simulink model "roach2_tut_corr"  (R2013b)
settings: Solver=VariableStepDiscrete  SolverMode=SingleTasking  StartTime=0.0  StopTime=100  RelTol=1e-3
undefined symbols (not defined in the file): add_latency, addr_width, Bit, bitfield, BitWidth, bram_latency, burst_size, casper_library_scopes, conv_latency, data_width, DelayLen, fan_latency, FFTSize, FFTStage, getfield, increment, led, Location, Lower, mult_latency, mux_latency, n_bits, n_bits_data, n_inputs, n_streams, n_taps, neg_latency, negate_latency, nsamples, pfb_size, pulse_len, reset_period, ROACH, ROACH2, snapshot, sx475t, sync_period, sync_period_bits, Upper, UseCounter, Width
libraries: xbsIndex_r4 x24444, casper_library_misc x73, xbsReplacements_r4 x34, casper_library_delays x14, xps_library x7
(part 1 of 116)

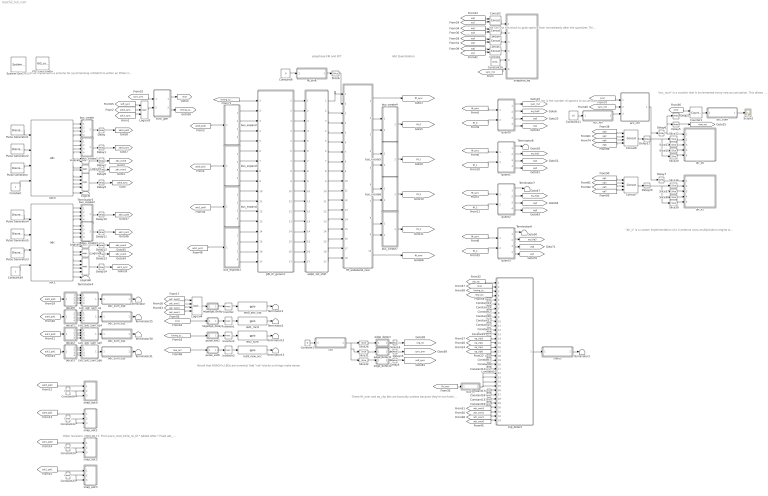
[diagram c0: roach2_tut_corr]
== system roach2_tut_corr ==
  note: This circuit implements a scheme for synchronizing a ROACH to within an FPGA clock of a second boundary using an external 1 pulse-per-second device. * A sync_arm command will cause the sync_gen to stop issuing sync pulses. * It will then ignore the next input trigger (1PPS), while sync is flushed through the DSP pipeline. * It will then lock onto the next trigger (1PPS) and issue syncs thereafter every sync_period clocks. * Need a multiple of (pfb_fir taps*LCM(FFT reorder orders) *fft bins/parallel inputs =) (4 * LCM(2,2,2,9) * 1024 / 4) = 18432) for sync_period for simulation * Trigger off either ADC's 1PPS inputs
  note: polyphase FIR and FFT
  note: "dir_x" is a custom implementation of a 4 antenna cross-multiplication engine which uses a multiplication core for each auto- and cross-correlation. Some BRAM space is wasted in this 1024 channel compile because the minimum shared BRAM size is 2048.
  note: "acc_num" is a counter that is incremented every new accumulation. This allows a computer to know when a new accumulation is available.
  note: acc_len is the number of spectra to accumulate.
  note: 4bit Quantisation
  note: Recall that ROACH's LEDs are inverted. Add "not" blocks so things make sense.
  note: Older revisions: 2009-08-17: From poco_mod_1024_no_fd * Added LEDs * Fixed adc_levels 2009-08-18: r310 * Changed dir_x numbering scheme * mods to adc_levels * added status register * EQ now per channel 2010-08-14: r313 * adc_sum_sq copied from kat-7 feng 2010-08-16: r314: * tidyup for workshop 2012-05-09: r315: * replaced FFT and PFB_FIR with new library ones * software register replacement 2013-08-16: r316: Updated for workshop. Ran DM's update_casper_blocks script Replaced all cross-multiplication modules with dsp48_cmults Replaced deprecated snap blocks Replaced FFT and FIR blocks for combined multi-input blocks.
  note: These fft_over and eq_clip bits are basically useless because they're non-latching. The chances of catching an actual overrange event from software is pretty small, unless they're continuously overranging.
  note: We can use this block to grab spectra from immediately after the quantizer. This will help determine what the correct quantizer EQ coefficients are
  " System Generator" : xbsIndex_r4/ System Generator  Tag=genX  xilinxfamily=virtex6  part=xc6vsx475t  speed=-1  package=ff1759  synthesis_tool=XST  clock_wrapper=Clock Enables  directory=./roach2_tut_corr/sysgen  proj_type=Project Navigator  Synth_file=XST Defaults  Impl_file=ISE Defaults  testbench=off  simulink_period=1  sysclk_period=5  dcm_input_clock_period=100  incr_netlist=off  trim_vbits=Everywhere in SubSystem  dbl_ovrd=According to Block Masks  core_generation=According to Block Masks  run_coregen=off  deprecated_control=off  eval_field=0  block_type=sysgen
  Concat{1..4} (4 alike) : xbsIndex_r4/Concat  num_inputs=2  dbl_ovrd=off  block_type=concat
  Concat6 : xbsIndex_r4/Concat  num_inputs=4  dbl_ovrd=off  block_type=concat
  Concat7 : xbsIndex_r4/Concat  num_inputs=4  dbl_ovrd=off  block_type=concat
  Constant : Constant  SampleTime=1/4
  Constant1 : Constant  Value=0
  Constant{2..5,7..8,10,12..21} (17 alike) : xbsIndex_r4/Constant  const=0  gui_display_data_type=Fixed-point  arith_type=Boolean  n_bits=1  bin_pt=0  preci_type=Single  exp_width=8  frac_width=24  explicit_period=on  period=1  equ=P=C  opselect=C  inp2=PCIN>>17  opr=+  inp1=P  carry=CIN  dbl_ovrd=off  block_type=constant
  Constant11 : Constant  Value=10
  Constant{6,22..24} (4 alike) : xbsIndex_r4/Constant  const=1  gui_display_data_type=Boolean  arith_type=Boolean  n_bits=16  bin_pt=14  preci_type=Single  exp_width=8  frac_width=24  explicit_period=on  period=1  equ=P=C  opselect=C  inp2=PCIN>>17  opr=+  inp1=P  carry=CIN  dbl_ovrd=off  block_type=constant
  Constant26 : xbsIndex_r4/Constant  const=0  gui_display_data_type=Boolean  arith_type=Boolean  n_bits=32  bin_pt=0  preci_type=Single  exp_width=8  frac_width=24  explicit_period=on  period=1  equ=P=C  opselect=C  inp2=PCIN>>17  opr=+  inp1=P  carry=CIN  dbl_ovrd=off  block_type=constant
  Constant39 : Constant  SampleTime=1/4
  Constant9 : Constant  Value=0
  Counter1 : xbsIndex_r4/Counter  cnt_type=Free Running  cnt_to=Inf  operation=Up  start_count=0  cnt_by_val=1  arith_type=Unsigned  n_bits=32  bin_pt=0  load_pin=off  rst=on  en=on  explicit_period=off  period=1  dbl_ovrd=off  use_behavioral_HDL=off  implementation=Fabric  use_rpm=on  block_type=counter
  Delay{,1..2,4..16} (16 alike) : xbsIndex_r4/Delay  rst=off  infoeditControl=Selection of Reset will increase slice count due to use of real FFs and instead of SRLs  en=off  latency=1  dbl_ovrd=off  reg_retiming=on  block_type=delay
  Delay20 : xbsIndex_r4/Delay  rst=off  infoeditControl=Selection of Reset will increase slice count due to use of real FFs and instead of SRLs  en=off  latency=2  dbl_ovrd=off  reg_retiming=on  block_type=delay
  Delay21 : xbsIndex_r4/Delay  rst=off  infoeditControl=Selection of Reset will increase slice count due to use of real FFs and instead of SRLs  en=off  latency=2  dbl_ovrd=off  reg_retiming=on  block_type=delay
  Delay3 : xbsIndex_r4/Delay  rst=off  infoeditControl=Selection of Reset will increase slice count due to use of real FFs and instead of SRLs  en=off  latency=2  dbl_ovrd=off  reg_retiming=on  block_type=delay
  Inverter{,1..3} (4 alike) : xbsIndex_r4/Inverter  en=off  latency=1  dbl_ovrd=off  block_type=inv
  Logical : xbsIndex_r4/Logical  logical_function=OR  inputs=4  en=off  latency=0  precision=Full  arith_type=Unsigned  n_bits=16  bin_pt=0  align_bp=on  dbl_ovrd=off  block_type=logical
  Logical{1..2,8..9} (4 alike) : xbsIndex_r4/Logical  logical_function=OR  inputs=2  en=off  latency=0  precision=Full  arith_type=Unsigned  n_bits=16  bin_pt=0  align_bp=on  dbl_ovrd=off  block_type=logical
  Logical3 : xbsIndex_r4/Logical  logical_function=OR  inputs=3  en=off  latency=0  precision=Full  arith_type=Unsigned  n_bits=16  bin_pt=0  align_bp=on  dbl_ovrd=off  block_type=logical
  Logical4 : xbsIndex_r4/Logical  logical_function=OR  inputs=4  en=off  latency=0  precision=Full  arith_type=Unsigned  n_bits=8  bin_pt=2  align_bp=on  dbl_ovrd=off  block_type=logical
  Logical6 : xbsIndex_r4/Logical  logical_function=OR  inputs=4  en=off  latency=0  precision=Full  arith_type=Unsigned  n_bits=16  bin_pt=0  align_bp=on  dbl_ovrd=off  block_type=logical
  Pulse Generator : DiscretePulseGenerator  Period=2^8  PhaseDelay=11  SampleTime=1/4
  Pulse Generator1 : DiscretePulseGenerator  Amplitude=0.75  Period=2^10  PhaseDelay=9+13+2^8  SampleTime=1/4
  Pulse Generator2 : DiscretePulseGenerator  Amplitude=0.5  Period=2^10  PhaseDelay=9+14+2^8  SampleTime=1/4
  Pulse Generator3 : DiscretePulseGenerator  Period=2^8  PhaseDelay=11  SampleTime=1/4
  Pulse Generator4 : DiscretePulseGenerator  Amplitude=0.75  Period=2^14  PhaseDelay=23+2^8  SampleTime=1/4
  Pulse Generator5 : DiscretePulseGenerator  Amplitude=0.5  Period=2^14  PhaseDelay=22+2^8  SampleTime=1/4
  Scope2 : Scope
  Slice12 : xbsIndex_r4/Slice  nbits=8  boolean_output=off  mode=Lower Bit Location + Width  bit1=0  base1=MSB of Input  bit0=24  base0=LSB of Input  dbl_ovrd=off  block_type=slice
  Slice13 : xbsIndex_r4/Slice  nbits=8  boolean_output=off  mode=Lower Bit Location + Width  bit1=0  base1=MSB of Input  bit0=16  base0=LSB of Input  dbl_ovrd=off  block_type=slice
  Slice15 : xbsIndex_r4/Slice  nbits=8  boolean_output=off  mode=Lower Bit Location + Width  bit1=0  base1=MSB of Input  bit0=8  base0=LSB of Input  dbl_ovrd=off  block_type=slice
  Slice20 : xbsIndex_r4/Slice  nbits=8  boolean_output=off  mode=Lower Bit Location + Width  bit1=0  base1=MSB of Input  bit0=0  base0=LSB of Input  dbl_ovrd=off  block_type=slice
  Slice26 : xbsIndex_r4/Slice  nbits=1  boolean_output=on  mode=Lower Bit Location + Width  bit1=0  base1=MSB of Input  bit0=16  base0=LSB of Input  dbl_ovrd=off  block_type=slice
  Slice31 : xbsIndex_r4/Slice  nbits=1  boolean_output=on  mode=Lower Bit Location + Width  bit1=0  base1=MSB of Input  bit0=17  base0=LSB of Input  dbl_ovrd=off  block_type=slice
  Slice32 : xbsIndex_r4/Slice  nbits=1  boolean_output=on  mode=Lower Bit Location + Width  bit1=0  base1=MSB of Input  bit0=18  base0=LSB of Input  dbl_ovrd=off  block_type=slice
  Slice36 : xbsIndex_r4/Slice  nbits=8  boolean_output=off  mode=Lower Bit Location + Width  bit1=0  base1=MSB of Input  bit0=24  base0=LSB of Input  dbl_ovrd=off  block_type=slice
  Slice37 : xbsIndex_r4/Slice  nbits=8  boolean_output=off  mode=Lower Bit Location + Width  bit1=0  base1=MSB of Input  bit0=16  base0=LSB of Input  dbl_ovrd=off  block_type=slice
  Slice38 : xbsIndex_r4/Slice  nbits=8  boolean_output=off  mode=Lower Bit Location + Width  bit1=0  base1=MSB of Input  bit0=8  base0=LSB of Input  dbl_ovrd=off  block_type=slice
  Slice39 : xbsIndex_r4/Slice  nbits=8  boolean_output=off  mode=Lower Bit Location + Width  bit1=0  base1=MSB of Input  bit0=0  base0=LSB of Input  dbl_ovrd=off  block_type=slice
  Slice6 : xbsIndex_r4/Slice  nbits=11  boolean_output=off  mode=Lower Bit Location + Width  bit1=0  base1=MSB of Input  bit0=0  base0=LSB of Input  dbl_ovrd=off  block_type=slice
  Terminator{,1..8,12..13,25,30..31} (14 alike) : Terminator
  XSG core config : xps_library/XSG_core_config  Tag=xps:xsg  hw_sys=ROACH2:sx475t  clk_src=adc0_clk  ROACH_clk_src=adc0_clk  ROACH2_clk_src=adc0_clk  MKDIG_clk_src=sys_clk  clk_rate=200  sample_period=1  synthesis_tool=XST
  a0p0_1st_shift : Subsystem
  acc_ctrl : Subsystem
  acc_len : Subsystem  Tag=xps:sw_reg  AncestorBlock=xps_library/software_register
  acc_num : Subsystem  Tag=xps:sw_reg  AncestorBlock=xps_library/software_register
  adc0 : xps_library/ADCs/adc  Tag=xps:adc  adc_brd=adc0  adc_clk_rate=800  adc_interleave=off  sample_period=1
  adc1 : xps_library/ADCs/adc  Tag=xps:adc  adc_brd=adc1  adc_clk_rate=800  adc_interleave=off  sample_period=1
  adc_sum_sq0 : Subsystem  Tag=xps:sw_reg  AncestorBlock=xps_library/software_register
  adc_sum_sq1 : Subsystem  Tag=xps:sw_reg  AncestorBlock=xps_library/software_register
  adc_sum_sq2 : Subsystem  Tag=xps:sw_reg  AncestorBlock=xps_library/software_register
  adc_sum_sq3 : Subsystem  Tag=xps:sw_reg  AncestorBlock=xps_library/software_register
  bus_create : Subsystem  AncestorBlock=casper_library_flow_control/bus_create
  bus_create1 : Subsystem  AncestorBlock=casper_library_flow_control/bus_create
  bus_create2 : Subsystem  AncestorBlock=casper_library_flow_control/bus_create
  bus_create3 : Subsystem  AncestorBlock=casper_library_flow_control/bus_create
  bus_create4 : Subsystem  AncestorBlock=casper_library_flow_control/bus_create
  bus_create5 : Subsystem  AncestorBlock=casper_library_flow_control/bus_create
  bus_create6 : Subsystem  AncestorBlock=casper_library_flow_control/bus_create
  bus_create7 : Subsystem  AncestorBlock=casper_library_flow_control/bus_create
  bus_expand : Subsystem  AncestorBlock=casper_library_flow_control/bus_expand
  bus_expand1 : Subsystem  AncestorBlock=casper_library_flow_control/bus_expand
  bus_expand2 : Subsystem  AncestorBlock=casper_library_flow_control/bus_expand
  bus_expand3 : Subsystem  AncestorBlock=casper_library_flow_control/bus_expand
  bus_or : Subsystem
  calc_adc_sum_sq : Subsystem
  calc_adc_sum_sq4 : Subsystem
  calc_adc_sum_sq5 : Subsystem
  calc_adc_sum_sq6 : Subsystem
  clip_detect : Subsystem
  ctrl : Subsystem  Tag=xps:sw_reg  AncestorBlock=xps_library/software_register
  decat0 : Subsystem
  decat1 : Subsystem
  decat2 : Subsystem
  decat3 : Subsystem
  dir_x0 : Subsystem
  dir_x1 : Subsystem
  edge_detect : Subsystem  AncestorBlock=casper_library_misc/edge_detect
  edge_detect1 : Subsystem  AncestorBlock=casper_library_misc/edge_detect
  edge_detect2 : Subsystem  AncestorBlock=casper_library_misc/edge_detect
  fft_shift : Subsystem  Tag=xps:sw_reg  AncestorBlock=xps_library/software_register
  fft_wideband_real : Subsystem  Tag=casper:fft_wideband_real  AncestorBlock=casper_library_ffts/fft_wideband_real
  led0_adc_clip : xps_library/gpio  Tag=xps:gpio  io_group=ROACH:led  io_dir=out  arith_type=Boolean  bitwidth=1  bin_pt=0  bit_index=0  sample_period=1  use_single_ended=off  use_ddr=off  reg_iob=on  reg_clk_phase=0  termination=None
  led1_mrst : xps_library/gpio  Tag=xps:gpio  io_group=ROACH:led  io_dir=out  arith_type=Boolean  bitwidth=1  bin_pt=0  bit_index=1  sample_period=1  use_single_ended=off  use_ddr=off  reg_iob=on  reg_clk_phase=0  termination=None
  led2_sync : xps_library/gpio  Tag=xps:gpio  io_group=ROACH:led  io_dir=out  arith_type=Boolean  bitwidth=1  bin_pt=0  bit_index=2  sample_period=1  use_single_ended=off  use_ddr=off  reg_iob=on  reg_clk_phase=0  termination=None
  led3_new_acc : xps_library/gpio  Tag=xps:gpio  io_group=ROACH:led  io_dir=out  arith_type=Unsigned  bitwidth=1  bin_pt=0  bit_index=3  sample_period=1  use_single_ended=off  use_ddr=off  reg_iob=on  reg_clk_phase=0  termination=None
  negedge_delay : Subsystem  AncestorBlock=casper_library_misc/negedge_delay
  negedge_delay1 : Subsystem  AncestorBlock=casper_library_misc/negedge_delay
  pfb_fir_generic : Subsystem  Tag=casper:pfb_fir_generic  AncestorBlock=casper_library_pfbs/pfb_fir_generic
  pulse_ext2 : Subsystem
  pulse_ext6 : Subsystem
  quant0 : Subsystem
  quant1 : Subsystem
  quant2 : Subsystem
  quant3 : Subsystem
  snap_adc0 : Subsystem  Tag=casper:snapshot  AncestorBlock=casper_library_scopes/snapshot
  snap_adc1 : Subsystem  Tag=casper:snapshot  AncestorBlock=casper_library_scopes/snapshot
  snap_adc2 : Subsystem  Tag=casper:snapshot  AncestorBlock=casper_library_scopes/snapshot
  snap_adc3 : Subsystem  Tag=casper:snapshot  AncestorBlock=casper_library_scopes/snapshot
  snapshot_eq : Subsystem  Tag=casper:bitsnap  AncestorBlock=casper_library_scopes/bitfield snapshot
  status : Subsystem  Tag=xps:sw_reg  AncestorBlock=xps_library/software_register
  sync_gen : Subsystem
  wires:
  adc0/16 -> Logical/4
  adc0/15 -> Logical/3
  adc0/14 -> Logical/2
  adc0/13 -> Logical/1
  Logical/1 -> Delay9/1
  adc0/9 -> Logical2/1
  adc0/10 -> Logical2/2
  adc0/11 -> Logical1/1
  adc0/12 -> Logical1/2
  Logical2/1 -> Delay2/1
  adc0/5 -> bus_create1/1(in1)
  adc0/6 -> bus_create1/2(in2)
  adc0/7 -> bus_create1/3(in3)
  adc0/8 -> bus_create1/4(in4)
  bus_create1/1(bus_out) -> Delay1/1
  adc0/1 -> bus_create/1(in1)
  adc0/2 -> bus_create/2(in2)
  adc0/3 -> bus_create/3(in3)
  adc0/4 -> bus_create/4(in4)
  bus_create/1(bus_out) -> Delay/1
  Pulse Generator/1 -> adc0/3
  Pulse Generator1/1 -> adc0/1
  Pulse Generator2/1 -> adc0/2
  Constant/1 -> adc0/4
  [adc0_sync] -> Logical3/2
  sync_gen/1(mrst) -> [mrst]
  sync_gen/2(sync) -> [timing_sync]
  Logical3/1 -> sync_gen/2(pps)
  [soft_sync] -> Logical3/1
  Constant9/1 -> fft_shift/1(sim_1)
  fft_shift/1(in_reg) -> Slice6/1
  [adc0_pol0] -> bus_expand/1(bus_in)
  adc1/16 -> Logical6/4
  adc1/15 -> Logical6/3
  adc1/14 -> Logical6/2
  adc1/13 -> Logical6/1
  Logical6/1 -> Delay14/1
  Pulse Generator3/1 -> adc1/3
  Pulse Generator4/1 -> adc1/1
  Pulse Generator5/1 -> adc1/2
  Constant39/1 -> adc1/4
  Logical1/1 -> Delay8/1
  quant0/1(sync_out) -> [sync_rnd]
  quant0/3(dout0) -> [eq0]
  quant0/4(dout1) -> [eq1]
  Constant11/1 -> acc_len/1(sim_1)
  acc_len/1(in_reg) -> acc_ctrl/3(acc_len)
  Concat6/1 -> Delay21/1
  Slice12/1 -> dir_x0/2(a)
  Slice13/1 -> dir_x0/3(b)
  Slice15/1 -> dir_x0/4(c)
  Slice20/1 -> dir_x0/5(d)
  Counter1/1 -> acc_num/1(out_reg)
  acc_ctrl/1(new_acc) -> Delay6/1, Delay7/1
  [mrst] -> acc_ctrl/1(mrst)
  Delay5/1 -> [new_acc]
  [sync_rnd] -> acc_ctrl/2(sync)
  acc_num/1(sim_out) -> Scope2/1
  Delay3/1 -> Counter1/2
  [mrst] -> Counter1/1
  Delay6/1 -> dir_x0/1(new_acc), Delay3/1, Delay5/1
  [eq0] -> Concat6/1
  [eq2] -> Concat6/2
  [eq4] -> Concat6/3
  [eq6] -> Concat6/4
  [eq1] -> Concat7/1
  [eq3] -> Concat7/2
  [eq5] -> Concat7/3
  [eq7] -> Concat7/4
  Delay20/1 -> Slice37/1, Slice38/1, Slice39/1, Slice36/1
  Slice36/1 -> dir_x1/2(a)
  Slice37/1 -> dir_x1/3(b)
  Slice38/1 -> dir_x1/4(c)
  Slice39/1 -> dir_x1/5(d)
  Concat7/1 -> Delay20/1
  Delay7/1 -> dir_x1/1(new_acc)
  [adc1_sync] -> Logical3/3
  Constant1/1 -> ctrl/1(sim_1)
  ctrl/1(in_reg) -> Slice26/1, Slice31/1, Slice32/1
  adc0/17 -> Terminator5/1
  adc1/17 -> Terminator4/1
  [clip_rst] -> clip_detect/1(rst)
  [adc_over3] -> clip_detect/30(In_03)
  [adc_over2] -> clip_detect/31(In_02)
  [adc_over1] -> clip_detect/32(In_01)
  [adc_over0] -> clip_detect/33(in_lsb)
  Constant16/1 -> clip_detect/29(In_04)
  Constant17/1 -> clip_detect/26(In_07)
  Constant18/1 -> clip_detect/27(In_06)
  Constant13/1 -> clip_detect/28(In_05)
  [mrst] -> clip_detect/2(in_msb_nr)
  [timing_sync] -> clip_detect/3(In_30_nr)
  [new_acc] -> clip_detect/4(In_29_nr)
  Constant14/1 -> clip_detect/5(In_28_nr)
  Constant19/1 -> clip_detect/6(In_27_nr)
  Constant2/1 -> clip_detect/7(In_26_nr)
  Constant20/1 -> clip_detect/8(In_25_nr)
  Constant21/1 -> clip_detect/9(In_24_nr)
  [eq_clip3] -> clip_detect/14(In_19)
  [eq_clip2] -> clip_detect/15(In_18)
  [eq_clip1] -> clip_detect/16(In_17)
  [eq_clip0] -> clip_detect/17(In_16)
  Constant7/1 -> clip_detect/18(In_15)
  Constant8/1 -> clip_detect/19(In_14)
  Constant10/1 -> clip_detect/20(In_13)
  Constant12/1 -> clip_detect/21(In_12)
  clip_detect/1(registered_out) -> status/1(out_reg)
  Slice26/1 -> edge_detect/1(in)
  [adc0_pol0] -> decat0/1(In1)
  Slice31/1 -> edge_detect1/1(in)
  Slice32/1 -> edge_detect2/1(in)
  edge_detect1/1(out) -> Delay15/1
  edge_detect/1(out) -> Delay16/1
  edge_detect2/1(out) -> Delay4/1
  [sync_arm] -> sync_gen/1(arm)
  Delay/1 -> [adc0_pol0]
  Delay1/1 -> [adc0_pol1]
  Delay2/1 -> [adc_over0]
  Delay8/1 -> [adc_over1]
  Delay9/1 -> [adc0_sync]
  Delay10/1 -> [adc1_pol0]
  Delay11/1 -> [adc1_pol1]
  Delay12/1 -> [adc_over2]
  Delay13/1 -> [adc_over3]
  Delay14/1 -> [adc1_sync]
  Delay21/1 -> Slice12/1, Slice13/1, Slice15/1, Slice20/1
  pulse_ext2/1(out) -> Inverter2/1
  [timing_sync] -> pulse_ext2/1(in)
  [mrst] -> negedge_delay1/1(in)
  pulse_ext6/1(out) -> Inverter3/1
  [new_acc] -> pulse_ext6/1(in)
  led0_adc_clip/1 -> Terminator1/1
  led1_mrst/1 -> Terminator2/1
  led2_sync/1 -> Terminator12/1
  led3_new_acc/1 -> Terminator13/1
  Logical4/1 -> negedge_delay/1(in)
  negedge_delay/1(out) -> Inverter/1
  [adc_over0] -> Logical4/1
  [adc_over1] -> Logical4/2
  [adc_over2] -> Logical4/3
  [adc_over3] -> Logical4/4
  negedge_delay1/1(out) -> Inverter1/1
  status/1(sim_out) -> Terminator3/1
  Constant15/1 -> clip_detect/10(In_23)
  Constant3/1 -> clip_detect/11(In_22)
  Constant4/1 -> clip_detect/12(In_21)
  Constant5/1 -> clip_detect/13(In_20)
  quant0/2(clip_out) -> [eq_clip0]
  quant1/1(sync_out) -> Terminator8/1
  quant1/3(dout0) -> [eq2]
  quant1/4(dout1) -> [eq3]
  quant1/2(clip_out) -> [eq_clip1]
  quant2/1(sync_out) -> Terminator7/1
  quant2/3(dout0) -> [eq4]
  quant2/2(clip_out) -> [eq_clip2]
  quant3/1(sync_out) -> Terminator6/1
  quant3/3(dout0) -> [eq6]
  quant3/4(dout1) -> [eq7]
  quant3/2(clip_out) -> [eq_clip3]
  Delay4/1 -> [soft_sync]
  Delay15/1 -> [sync_arm]
  Delay16/1 -> [clip_rst]
  Inverter/1 -> led0_adc_clip/1
  Inverter1/1 -> led1_mrst/1
  Inverter2/1 -> led2_sync/1
  Inverter3/1 -> led3_new_acc/1
  adc1/9 -> Logical9/1
  adc1/10 -> Logical9/2
  adc1/11 -> Logical8/1
  adc1/12 -> Logical8/2
  Logical9/1 -> Delay12/1
  Logical8/1 -> Delay13/1
  adc1/5 -> bus_create3/1(in1)
  adc1/6 -> bus_create3/2(in2)
  adc1/7 -> bus_create3/3(in3)
  adc1/8 -> bus_create3/4(in4)
  bus_create3/1(bus_out) -> Delay11/1
  adc1/1 -> bus_create2/1(in1)
  adc1/2 -> bus_create2/2(in2)
  adc1/3 -> bus_create2/3(in3)
  adc1/4 -> bus_create2/4(in4)
  bus_create2/1(bus_out) -> Delay10/1
  calc_adc_sum_sq/1(sum_sq) -> adc_sum_sq0/1(out_reg)
  decat0/1(Out1) -> calc_adc_sum_sq/1(In1)
  decat0/2(Out2) -> calc_adc_sum_sq/2(In2)
  decat0/3(Out3) -> calc_adc_sum_sq/3(In3)
  decat0/4(Out4) -> calc_adc_sum_sq/4(In4)
  adc_sum_sq0/1(sim_out) -> Terminator/1
  calc_adc_sum_sq4/1(sum_sq) -> adc_sum_sq1/1(out_reg)
  decat1/1(Out1) -> calc_adc_sum_sq4/1(In1)
  decat1/2(Out2) -> calc_adc_sum_sq4/2(In2)
  decat1/3(Out3) -> calc_adc_sum_sq4/3(In3)
  decat1/4(Out4) -> calc_adc_sum_sq4/4(In4)
  adc_sum_sq1/1(sim_out) -> Terminator25/1
  calc_adc_sum_sq5/1(sum_sq) -> adc_sum_sq2/1(out_reg)
  decat2/1(Out1) -> calc_adc_sum_sq5/1(In1)
  decat2/2(Out2) -> calc_adc_sum_sq5/2(In2)
  decat2/3(Out3) -> calc_adc_sum_sq5/3(In3)
  decat2/4(Out4) -> calc_adc_sum_sq5/4(In4)
  adc_sum_sq2/1(sim_out) -> Terminator30/1
  calc_adc_sum_sq6/1(sum_sq) -> adc_sum_sq3/1(out_reg)
  decat3/1(Out1) -> calc_adc_sum_sq6/1(In1)
  decat3/2(Out2) -> calc_adc_sum_sq6/2(In2)
  decat3/3(Out3) -> calc_adc_sum_sq6/3(In3)
  decat3/4(Out4) -> calc_adc_sum_sq6/4(In4)
  adc_sum_sq3/1(sim_out) -> Terminator31/1
  [adc0_pol1] -> decat1/1(In1)
  [adc1_pol0] -> decat2/1(In1)
  [adc1_pol1] -> decat3/1(In1)
  quant2/4(dout1) -> [eq5]
  [fft_over] -> bus_or/1(In1)
  Slice6/1 -> fft_wideband_real/2(shift)
  fft_wideband_real/10(of) -> [fft_over]
  a0p0_1st_shift/1(sync_out) -> fft_wideband_real/1(sync)
  a0p0_1st_shift/14(dout13) -> fft_wideband_real/15(in30)
  a0p0_1st_shift/10(dout9) -> fft_wideband_real/11(in20)
  a0p0_1st_shift/11(dout10) -> fft_wideband_real/12(in21)
  a0p0_1st_shift/12(dout11) -> fft_wideband_real/13(in22)
  a0p0_1st_shift/13(dout12) -> fft_wideband_real/14(in23)
  a0p0_1st_shift/15(dout14) -> fft_wideband_real/16(in31)
  a0p0_1st_shift/16(dout15) -> fft_wideband_real/17(in32)
  a0p0_1st_shift/17(dout16) -> fft_wideband_real/18(in33)
  a0p0_1st_shift/6(dout5) -> fft_wideband_real/7(in10)
  a0p0_1st_shift/7(dout6) -> fft_wideband_real/8(in11)
  a0p0_1st_shift/8(dout7) -> fft_wideband_real/9(in12)
  a0p0_1st_shift/9(dout8) -> fft_wideband_real/10(in13)
  a0p0_1st_shift/2(dout1) -> fft_wideband_real/3(in00)
  a0p0_1st_shift/3(dout2) -> fft_wideband_real/4(in01)
  a0p0_1st_shift/5(dout4) -> fft_wideband_real/6(in03)
  a0p0_1st_shift/4(dout3) -> fft_wideband_real/5(in02)
  [adc0_pol1] -> bus_expand1/1(bus_in)
  [adc1_pol0] -> bus_expand2/1(bus_in)
  [adc1_pol1] -> bus_expand3/1(bus_in)
  pfb_fir_generic/1(sync_out) -> a0p0_1st_shift/1(sync_in)
  pfb_fir_generic/2(pol0_out0) -> a0p0_1st_shift/2(din1)
  pfb_fir_generic/6(pol1_out0) -> a0p0_1st_shift/6(din5)
  pfb_fir_generic/7(pol1_out1) -> a0p0_1st_shift/7(din6)
  pfb_fir_generic/8(pol1_out2) -> a0p0_1st_shift/8(din7)
  pfb_fir_generic/14(pol3_out0) -> a0p0_1st_shift/14(din13)
  pfb_fir_generic/3(pol0_out1) -> a0p0_1st_shift/3(din2)
  pfb_fir_generic/5(pol0_out3) -> a0p0_1st_shift/5(din4)
  pfb_fir_generic/10(pol2_out0) -> a0p0_1st_shift/10(din9)
  pfb_fir_generic/13(pol2_out3) -> a0p0_1st_shift/13(din12)
  pfb_fir_generic/15(pol3_out1) -> a0p0_1st_shift/15(din14)
  pfb_fir_generic/12(pol2_out2) -> a0p0_1st_shift/12(din11)
  pfb_fir_generic/4(pol0_out2) -> a0p0_1st_shift/4(din3)
  pfb_fir_generic/11(pol2_out1) -> a0p0_1st_shift/11(din10)
  pfb_fir_generic/16(pol3_out2) -> a0p0_1st_shift/16(din15)
  pfb_fir_generic/17(pol3_out3) -> a0p0_1st_shift/17(din16)
  pfb_fir_generic/9(pol1_out3) -> a0p0_1st_shift/9(din8)
  [timing_sync] -> pfb_fir_generic/1(sync)
  bus_expand/2(out3) -> pfb_fir_generic/3(pol0_in1)
  bus_expand/3(out2) -> pfb_fir_generic/4(pol0_in2)
  bus_expand/4(lsb_out1) -> pfb_fir_generic/5(pol0_in3)
  bus_expand/1(msb_out4) -> pfb_fir_generic/2(pol0_in0)
  bus_expand1/1(msb_out4) -> pfb_fir_generic/6(pol1_in0)
  bus_expand1/2(out3) -> pfb_fir_generic/7(pol1_in1)
  bus_expand1/3(out2) -> pfb_fir_generic/8(pol1_in2)
  bus_expand1/4(lsb_out1) -> pfb_fir_generic/9(pol1_in3)
  bus_expand2/2(out3) -> pfb_fir_generic/11(pol2_in1)
  bus_expand2/3(out2) -> pfb_fir_generic/12(pol2_in2)
  bus_expand2/4(lsb_out1) -> pfb_fir_generic/13(pol2_in3)
  bus_expand2/1(msb_out4) -> pfb_fir_generic/10(pol2_in0)
  bus_expand3/2(out3) -> pfb_fir_generic/15(pol3_in1)
  bus_expand3/1(msb_out4) -> pfb_fir_generic/14(pol3_in0)
  bus_expand3/3(out2) -> pfb_fir_generic/16(pol3_in2)
  bus_expand3/4(lsb_out1) -> pfb_fir_generic/17(pol3_in3)
  bus_or/1(Out1) -> clip_detect/22(In_11), clip_detect/23(In_10), clip_detect/24(In_09), clip_detect/25(In_08)
  fft_wideband_real/2(out00) -> bus_create4/1(in1)
  fft_wideband_real/3(out01) -> bus_create4/2(in2)
  fft_wideband_real/1(sync_out) -> [fft_sync]
  bus_create4/1(bus_out) -> [fft_0]
  [fft_sync] -> quant0/1(sync)
  [fft_sync] -> quant1/1(sync)
  [fft_sync] -> quant2/1(sync)
  [fft_sync] -> quant3/1(sync)
  [fft_0] -> quant0/2(din)
  [fft_1] -> quant1/2(din)
  [fft_2] -> quant2/2(din)
  [fft_3] -> quant3/2(din)
  Constant6/1 -> snap_adc0/3(trig), snap_adc0/2(we)
  Constant22/1 -> snap_adc1/2(we), snap_adc1/3(trig)
  Constant24/1 -> snap_adc2/2(we), snap_adc2/3(trig)
  Constant23/1 -> snap_adc3/3(trig), snap_adc3/2(we)
  [adc0_pol0] -> snap_adc0/1(din)
  [adc0_pol1] -> snap_adc1/1(din)
  [adc1_pol0] -> snap_adc2/1(din)
  [adc1_pol1] -> snap_adc3/1(din)
  fft_wideband_real/5(out11) -> bus_create5/2(in2)
  fft_wideband_real/4(out10) -> bus_create5/1(in1)
  bus_create5/1(bus_out) -> [fft_1]
  fft_wideband_real/7(out21) -> bus_create6/2(in2)
  fft_wideband_real/6(out20) -> bus_create6/1(in1)
  bus_create6/1(bus_out) -> [fft_2]
  fft_wideband_real/9(out31) -> bus_create7/2(in2)
  fft_wideband_real/8(out30) -> bus_create7/1(in1)
  bus_create7/1(bus_out) -> [fft_3]
  Constant26/1 -> snapshot_eq/5(we)
  [sync_rnd] -> snapshot_eq/6(trig)
  Concat2/1 -> snapshot_eq/1(in_quant0)
  Concat4/1 -> snapshot_eq/2(in_quant1)
  Concat3/1 -> snapshot_eq/3(in_quant2)
  [eq0] -> Concat2/1
  [eq1] -> Concat2/2
  [eq4] -> Concat3/1
  [eq2] -> Concat4/1
  [eq3] -> Concat4/2
  [eq5] -> Concat3/2
  Concat1/1 -> snapshot_eq/4(in_quant3)
  [eq6] -> Concat1/1
  [eq7] -> Concat1/2

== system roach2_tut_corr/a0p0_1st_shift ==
  sync_in : Inport
  din1 : Inport  Port=2
  din2 : Inport  Port=3
  din3 : Inport  Port=4
  din4 : Inport  Port=5
  din5 : Inport  Port=6
  din6 : Inport  Port=7
  din7 : Inport  Port=8
  din8 : Inport  Port=9
  din9 : Inport  Port=10
  din10 : Inport  Port=11
  din11 : Inport  Port=12
  din12 : Inport  Port=13
  din13 : Inport  Port=14
  din14 : Inport  Port=15
  din15 : Inport  Port=16
  din16 : Inport  Port=17
  Delay : xbsIndex_r4/Delay  rst=off  infoeditControl=Selection of Reset will increase slice count due to use of real FFs and instead of SRLs  en=off  latency=latency  dbl_ovrd=off  reg_retiming=off  block_type=delay
  Shift{1..16} (16 alike) : xbsIndex_r4/Shift  shift_dir=Right  shift_bits=shift  en=off  latency=latency  precision=Full  arith_type="Signed  (2's comp)"  n_bits=16  bin_pt=14  quantization=Truncate  overflow=Wrap  dbl_ovrd=off  block_type=shift
  sync_out : Outport
  dout1 : Outport  Port=2
  dout2 : Outport  Port=3
  dout3 : Outport  Port=4
  dout4 : Outport  Port=5
  dout5 : Outport  Port=6
  dout6 : Outport  Port=7
  dout7 : Outport  Port=8
  dout8 : Outport  Port=9
  dout9 : Outport  Port=10
  dout10 : Outport  Port=11
  dout11 : Outport  Port=12
  dout12 : Outport  Port=13
  dout13 : Outport  Port=14
  dout14 : Outport  Port=15
  dout15 : Outport  Port=16
  dout16 : Outport  Port=17
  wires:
  din1/1 -> Shift3/1
  Shift3/1 -> dout1/1
  din2/1 -> Shift1/1
  Shift1/1 -> dout2/1
  din3/1 -> Shift4/1
  Shift4/1 -> dout3/1
  din4/1 -> Shift2/1
  Shift2/1 -> dout4/1
  sync_in/1 -> Delay/1
  Delay/1 -> sync_out/1
  din5/1 -> Shift7/1
  Shift7/1 -> dout5/1
  din6/1 -> Shift5/1
  Shift5/1 -> dout6/1
  din7/1 -> Shift8/1
  Shift8/1 -> dout7/1
  din8/1 -> Shift6/1
  Shift6/1 -> dout8/1
  din9/1 -> Shift11/1
  Shift11/1 -> dout9/1
  din10/1 -> Shift9/1
  Shift9/1 -> dout10/1
  din11/1 -> Shift12/1
  Shift12/1 -> dout11/1
  din12/1 -> Shift10/1
  Shift10/1 -> dout12/1
  din13/1 -> Shift15/1
  Shift15/1 -> dout13/1
  din14/1 -> Shift13/1
  Shift13/1 -> dout14/1
  din15/1 -> Shift14/1
  Shift14/1 -> dout15/1
  din16/1 -> Shift16/1
  Shift16/1 -> dout16/1

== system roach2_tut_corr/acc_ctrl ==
  mrst : Inport
  sync : Inport  Port=2
  acc_len : Inport  Port=3
  Delay : xbsIndex_r4/Delay  rst=off  infoeditControl=Selection of Reset will increase slice count due to use of real FFs and instead of SRLs  en=off  latency=1  dbl_ovrd=off  reg_retiming=on  block_type=delay
  Logical : xbsIndex_r4/Logical  logical_function=OR  inputs=2  en=off  latency=0  precision=Full  arith_type=Unsigned  n_bits=8  bin_pt=2  align_bp=on  dbl_ovrd=off  block_type=logical
  Register : xbsIndex_r4/Register  init=0  rst=on  en=on  dbl_ovrd=off  block_type=register
  Relational5 : xbsIndex_r4/Relational  mode=a>=b  en=off  latency=0  dbl_ovrd=off  block_type=relational
  Shift : xbsIndex_r4/Shift  shift_dir=Left  shift_bits=chan_bits  en=off  latency=0  precision=Full  arith_type="Signed  (2's comp)"  n_bits=8  bin_pt=2  quantization=Truncate  overflow=Wrap  dbl_ovrd=off  block_type=shift
  cntr : xbsIndex_r4/Counter  cnt_type=Free Running  cnt_to=Inf  operation=Up  start_count=1  cnt_by_val=1  arith_type=Unsigned  n_bits=32  bin_pt=0  load_pin=off  rst=on  en=off  explicit_period=on  period=1  dbl_ovrd=off  use_behavioral_HDL=off  implementation=Fabric  use_rpm=on  block_type=counter
  edge_detect : Subsystem  AncestorBlock=casper_library_misc/edge_detect
  edge_detect1 : Subsystem  AncestorBlock=casper_library_misc/edge_detect
  edge_detect2 : Subsystem  AncestorBlock=casper_library_misc/edge_detect
  new_acc : Outport
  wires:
  Relational5/1 -> Logical/2, edge_detect2/1(in)
  acc_len/1 -> Shift/1
  edge_detect2/1(out) -> new_acc/1
  Logical/1 -> cntr/1
  Register/1 -> edge_detect1/1(in)
  edge_detect/1(out) -> Register/2
  edge_detect1/1(out) -> Logical/1
  Delay/1 -> Relational5/2
  Shift/1 -> Delay/1
  cntr/1 -> Relational5/1
  mrst/1 -> edge_detect/1(in)
  sync/1 -> Register/1, Register/3

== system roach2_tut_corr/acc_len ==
  sim_1 : Inport
  io_delay : xbsIndex_r4/Delay  rst=off  infoeditControl=Selection of Reset will increase slice count due to use of real FFs and instead of SRLs  en=off  latency=0  dbl_ovrd=off  reg_retiming=on  block_type=delay
  reint1 : xbsIndex_r4/Reinterpret  force_arith_type=on  arith_type=Unsigned  force_bin_pt=on  bin_pt=0  block_type=reinterpret
  roach2_tut_corr_acc_len_user_data_out : xbsIndex_r4/Gateway In  gui_display_data_type=Fixed-point  arith_type=Unsigned  n_bits=32  bin_pt=0  preci_type=Single  exp_width=8  frac_width=24  quantization="Round  (unbiased: +/- Inf)"  overflow=Saturate  period=1  dbl_ovrd=off  timing_constraint=None  locs_specified=off  LOCs={}  UseAsADC=off  ADCChannel='1'  inherit_from_input=off  hdl_port=on  block_type=gatewayin
  slice_reg : xbsIndex_r4/Slice  nbits=32  boolean_output=off  mode=Lower Bit Location + Width  bit1=0  base1=MSB of Input  bit0=0  base0=LSB of Input  dbl_ovrd=off  block_type=slice
  in_reg : Outport
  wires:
  roach2_tut_corr_acc_len_user_data_out/1 -> io_delay/1
  sim_1/1 -> roach2_tut_corr_acc_len_user_data_out/1
  io_delay/1 -> slice_reg/1
  slice_reg/1 -> reint1/1
  reint1/1 -> in_reg/1

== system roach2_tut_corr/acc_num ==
  out_reg : Inport
  assert_reg : xbsIndex_r4/Assert  assert_type=on  type_source=Explicitly  gui_display_data_type=Fixed-point  arith_type=Unsigned  n_bits=32  bin_pt=0  preci_type=Single  exp_width=8  frac_width=24  assert_rate=off  rate_source=Explicitly  period=1  output_port=on  block_type=assert
  cast_gw : xbsIndex_r4/Convert  gui_display_data_type=Fixed-point  arith_type=Unsigned  n_bits=32  bin_pt=0  float_type=Single  exp_bits=8  fraction_bits=24  quantization=Truncate  overflow=Wrap  en=off  latency=0  dbl_ovrd=off  pipeline=off  block_type=convert
  io_delay : xbsIndex_r4/Delay  rst=off  infoeditControl=Selection of Reset will increase slice count due to use of real FFs and instead of SRLs  en=off  latency=0  dbl_ovrd=off  reg_retiming=on  block_type=delay
  reint1 : xbsIndex_r4/Reinterpret  force_arith_type=on  arith_type=Unsigned  force_bin_pt=on  bin_pt=0  block_type=reinterpret
  roach2_tut_corr_acc_num_user_data_in : xbsIndex_r4/Gateway Out  inherit_from_input=off  hdl_port=on  timing_constraint=None  locs_specified=off  LOCs={}  UseAsDAC=off  DACChannel='1'  block_type=gatewayout
  sim_out : Outport
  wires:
  io_delay/1 -> cast_gw/1
  cast_gw/1 -> roach2_tut_corr_acc_num_user_data_in/1
  roach2_tut_corr_acc_num_user_data_in/1 -> sim_out/1
  out_reg/1 -> assert_reg/1
  assert_reg/1 -> reint1/1
  reint1/1 -> io_delay/1

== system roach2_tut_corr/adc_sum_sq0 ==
  out_reg : Inport
  assert_reg : xbsIndex_r4/Assert  assert_type=on  type_source=Explicitly  gui_display_data_type=Fixed-point  arith_type=Unsigned  n_bits=32  bin_pt=0  preci_type=Single  exp_width=8  frac_width=24  assert_rate=off  rate_source=Explicitly  period=1  output_port=on  block_type=assert
  cast_gw : xbsIndex_r4/Convert  gui_display_data_type=Fixed-point  arith_type=Unsigned  n_bits=32  bin_pt=0  float_type=Single  exp_bits=8  fraction_bits=24  quantization=Truncate  overflow=Wrap  en=off  latency=0  dbl_ovrd=off  pipeline=off  block_type=convert
  io_delay : xbsIndex_r4/Delay  rst=off  infoeditControl=Selection of Reset will increase slice count due to use of real FFs and instead of SRLs  en=off  latency=0  dbl_ovrd=off  reg_retiming=on  block_type=delay
  reint1 : xbsIndex_r4/Reinterpret  force_arith_type=on  arith_type=Unsigned  force_bin_pt=on  bin_pt=0  block_type=reinterpret
  roach2_tut_corr_adc_sum_sq0_user_data_in : xbsIndex_r4/Gateway Out  inherit_from_input=off  hdl_port=on  timing_constraint=None  locs_specified=off  LOCs={}  UseAsDAC=off  DACChannel='1'  block_type=gatewayout
  sim_out : Outport
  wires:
  io_delay/1 -> cast_gw/1
  cast_gw/1 -> roach2_tut_corr_adc_sum_sq0_user_data_in/1
  roach2_tut_corr_adc_sum_sq0_user_data_in/1 -> sim_out/1
  out_reg/1 -> assert_reg/1
  assert_reg/1 -> reint1/1
  reint1/1 -> io_delay/1

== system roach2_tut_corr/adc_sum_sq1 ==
  out_reg : Inport
  assert_reg : xbsIndex_r4/Assert  assert_type=on  type_source=Explicitly  gui_display_data_type=Fixed-point  arith_type=Unsigned  n_bits=32  bin_pt=0  preci_type=Single  exp_width=8  frac_width=24  assert_rate=off  rate_source=Explicitly  period=1  output_port=on  block_type=assert
  cast_gw : xbsIndex_r4/Convert  gui_display_data_type=Fixed-point  arith_type=Unsigned  n_bits=32  bin_pt=0  float_type=Single  exp_bits=8  fraction_bits=24  quantization=Truncate  overflow=Wrap  en=off  latency=0  dbl_ovrd=off  pipeline=off  block_type=convert
  io_delay : xbsIndex_r4/Delay  rst=off  infoeditControl=Selection of Reset will increase slice count due to use of real FFs and instead of SRLs  en=off  latency=0  dbl_ovrd=off  reg_retiming=on  block_type=delay
  reint1 : xbsIndex_r4/Reinterpret  force_arith_type=on  arith_type=Unsigned  force_bin_pt=on  bin_pt=0  block_type=reinterpret
  roach2_tut_corr_adc_sum_sq1_user_data_in : xbsIndex_r4/Gateway Out  inherit_from_input=off  hdl_port=on  timing_constraint=None  locs_specified=off  LOCs={}  UseAsDAC=off  DACChannel='1'  block_type=gatewayout
  sim_out : Outport
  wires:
  io_delay/1 -> cast_gw/1
  cast_gw/1 -> roach2_tut_corr_adc_sum_sq1_user_data_in/1
  roach2_tut_corr_adc_sum_sq1_user_data_in/1 -> sim_out/1
  out_reg/1 -> assert_reg/1
  assert_reg/1 -> reint1/1
  reint1/1 -> io_delay/1

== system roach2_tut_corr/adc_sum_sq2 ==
  out_reg : Inport
  assert_reg : xbsIndex_r4/Assert  assert_type=on  type_source=Explicitly  gui_display_data_type=Fixed-point  arith_type=Unsigned  n_bits=32  bin_pt=0  preci_type=Single  exp_width=8  frac_width=24  assert_rate=off  rate_source=Explicitly  period=1  output_port=on  block_type=assert
  cast_gw : xbsIndex_r4/Convert  gui_display_data_type=Fixed-point  arith_type=Unsigned  n_bits=32  bin_pt=0  float_type=Single  exp_bits=8  fraction_bits=24  quantization=Truncate  overflow=Wrap  en=off  latency=0  dbl_ovrd=off  pipeline=off  block_type=convert
  io_delay : xbsIndex_r4/Delay  rst=off  infoeditControl=Selection of Reset will increase slice count due to use of real FFs and instead of SRLs  en=off  latency=0  dbl_ovrd=off  reg_retiming=on  block_type=delay
  reint1 : xbsIndex_r4/Reinterpret  force_arith_type=on  arith_type=Unsigned  force_bin_pt=on  bin_pt=0  block_type=reinterpret
  roach2_tut_corr_adc_sum_sq2_user_data_in : xbsIndex_r4/Gateway Out  inherit_from_input=off  hdl_port=on  timing_constraint=None  locs_specified=off  LOCs={}  UseAsDAC=off  DACChannel='1'  block_type=gatewayout
  sim_out : Outport
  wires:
  io_delay/1 -> cast_gw/1
  cast_gw/1 -> roach2_tut_corr_adc_sum_sq2_user_data_in/1
  roach2_tut_corr_adc_sum_sq2_user_data_in/1 -> sim_out/1
  out_reg/1 -> assert_reg/1
  assert_reg/1 -> reint1/1
  reint1/1 -> io_delay/1

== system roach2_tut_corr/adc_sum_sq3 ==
  out_reg : Inport
  assert_reg : xbsIndex_r4/Assert  assert_type=on  type_source=Explicitly  gui_display_data_type=Fixed-point  arith_type=Unsigned  n_bits=32  bin_pt=0  preci_type=Single  exp_width=8  frac_width=24  assert_rate=off  rate_source=Explicitly  period=1  output_port=on  block_type=assert
  cast_gw : xbsIndex_r4/Convert  gui_display_data_type=Fixed-point  arith_type=Unsigned  n_bits=32  bin_pt=0  float_type=Single  exp_bits=8  fraction_bits=24  quantization=Truncate  overflow=Wrap  en=off  latency=0  dbl_ovrd=off  pipeline=off  block_type=convert
  io_delay : xbsIndex_r4/Delay  rst=off  infoeditControl=Selection of Reset will increase slice count due to use of real FFs and instead of SRLs  en=off  latency=0  dbl_ovrd=off  reg_retiming=on  block_type=delay
  reint1 : xbsIndex_r4/Reinterpret  force_arith_type=on  arith_type=Unsigned  force_bin_pt=on  bin_pt=0  block_type=reinterpret
  roach2_tut_corr_adc_sum_sq3_user_data_in : xbsIndex_r4/Gateway Out  inherit_from_input=off  hdl_port=on  timing_constraint=None  locs_specified=off  LOCs={}  UseAsDAC=off  DACChannel='1'  block_type=gatewayout
  sim_out : Outport
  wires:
  io_delay/1 -> cast_gw/1
  cast_gw/1 -> roach2_tut_corr_adc_sum_sq3_user_data_in/1
  roach2_tut_corr_adc_sum_sq3_user_data_in/1 -> sim_out/1
  out_reg/1 -> assert_reg/1
  assert_reg/1 -> reint1/1
  reint1/1 -> io_delay/1

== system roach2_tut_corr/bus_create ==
  in1 : Inport
  in2 : Inport  Port=2
  in3 : Inport  Port=3
  in4 : Inport  Port=4
  concatenate : xbsIndex_r4/Concat  num_inputs=4  dbl_ovrd=off  block_type=concat
  reinterpret{1..4} (4 alike) : xbsIndex_r4/Reinterpret  force_arith_type=on  arith_type=Unsigned  force_bin_pt=on  bin_pt=0  block_type=reinterpret
  bus_out : Outport
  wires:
  concatenate/1 -> bus_out/1
  in1/1 -> reinterpret1/1
  reinterpret1/1 -> concatenate/1
  in2/1 -> reinterpret2/1
  reinterpret2/1 -> concatenate/2
  in3/1 -> reinterpret3/1
  reinterpret3/1 -> concatenate/3
  in4/1 -> reinterpret4/1
  reinterpret4/1 -> concatenate/4

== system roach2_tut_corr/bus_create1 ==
  in1 : Inport
  in2 : Inport  Port=2
  in3 : Inport  Port=3
  in4 : Inport  Port=4
  concatenate : xbsIndex_r4/Concat  num_inputs=4  dbl_ovrd=off  block_type=concat
  reinterpret{1..4} (4 alike) : xbsIndex_r4/Reinterpret  force_arith_type=on  arith_type=Unsigned  force_bin_pt=on  bin_pt=0  block_type=reinterpret
  bus_out : Outport
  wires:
  concatenate/1 -> bus_out/1
  in1/1 -> reinterpret1/1
  reinterpret1/1 -> concatenate/1
  in2/1 -> reinterpret2/1
  reinterpret2/1 -> concatenate/2
  in3/1 -> reinterpret3/1
  reinterpret3/1 -> concatenate/3
  in4/1 -> reinterpret4/1
  reinterpret4/1 -> concatenate/4

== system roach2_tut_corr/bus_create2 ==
  in1 : Inport
  in2 : Inport  Port=2
  in3 : Inport  Port=3
  in4 : Inport  Port=4
  concatenate : xbsIndex_r4/Concat  num_inputs=4  dbl_ovrd=off  block_type=concat
  reinterpret{1..4} (4 alike) : xbsIndex_r4/Reinterpret  force_arith_type=on  arith_type=Unsigned  force_bin_pt=on  bin_pt=0  block_type=reinterpret
  bus_out : Outport
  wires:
  concatenate/1 -> bus_out/1
  in1/1 -> reinterpret1/1
  reinterpret1/1 -> concatenate/1
  in2/1 -> reinterpret2/1
  reinterpret2/1 -> concatenate/2
  in3/1 -> reinterpret3/1
  reinterpret3/1 -> concatenate/3
  in4/1 -> reinterpret4/1
  reinterpret4/1 -> concatenate/4

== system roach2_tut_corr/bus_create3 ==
  in1 : Inport
  in2 : Inport  Port=2
  in3 : Inport  Port=3
  in4 : Inport  Port=4
  concatenate : xbsIndex_r4/Concat  num_inputs=4  dbl_ovrd=off  block_type=concat
  reinterpret{1..4} (4 alike) : xbsIndex_r4/Reinterpret  force_arith_type=on  arith_type=Unsigned  force_bin_pt=on  bin_pt=0  block_type=reinterpret
  bus_out : Outport
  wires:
  concatenate/1 -> bus_out/1
  in1/1 -> reinterpret1/1
  reinterpret1/1 -> concatenate/1
  in2/1 -> reinterpret2/1
  reinterpret2/1 -> concatenate/2
  in3/1 -> reinterpret3/1
  reinterpret3/1 -> concatenate/3
  in4/1 -> reinterpret4/1
  reinterpret4/1 -> concatenate/4

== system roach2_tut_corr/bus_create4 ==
  in1 : Inport
  in2 : Inport  Port=2
  concatenate : xbsIndex_r4/Concat  num_inputs=2  dbl_ovrd=off  block_type=concat
  reinterpret1 : xbsIndex_r4/Reinterpret  force_arith_type=on  arith_type=Unsigned  force_bin_pt=on  bin_pt=0  block_type=reinterpret
  reinterpret2 : xbsIndex_r4/Reinterpret  force_arith_type=on  arith_type=Unsigned  force_bin_pt=on  bin_pt=0  block_type=reinterpret
  bus_out : Outport
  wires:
  concatenate/1 -> bus_out/1
  in1/1 -> reinterpret1/1
  reinterpret1/1 -> concatenate/1
  in2/1 -> reinterpret2/1
  reinterpret2/1 -> concatenate/2

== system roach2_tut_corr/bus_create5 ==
  in1 : Inport
  in2 : Inport  Port=2
  concatenate : xbsIndex_r4/Concat  num_inputs=2  dbl_ovrd=off  block_type=concat
  reinterpret1 : xbsIndex_r4/Reinterpret  force_arith_type=on  arith_type=Unsigned  force_bin_pt=on  bin_pt=0  block_type=reinterpret
  reinterpret2 : xbsIndex_r4/Reinterpret  force_arith_type=on  arith_type=Unsigned  force_bin_pt=on  bin_pt=0  block_type=reinterpret
  bus_out : Outport
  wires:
  concatenate/1 -> bus_out/1
  in1/1 -> reinterpret1/1
  reinterpret1/1 -> concatenate/1
  in2/1 -> reinterpret2/1
  reinterpret2/1 -> concatenate/2

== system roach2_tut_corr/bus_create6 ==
  in1 : Inport
  in2 : Inport  Port=2
  concatenate : xbsIndex_r4/Concat  num_inputs=2  dbl_ovrd=off  block_type=concat
  reinterpret1 : xbsIndex_r4/Reinterpret  force_arith_type=on  arith_type=Unsigned  force_bin_pt=on  bin_pt=0  block_type=reinterpret
  reinterpret2 : xbsIndex_r4/Reinterpret  force_arith_type=on  arith_type=Unsigned  force_bin_pt=on  bin_pt=0  block_type=reinterpret
  bus_out : Outport
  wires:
  concatenate/1 -> bus_out/1
  in1/1 -> reinterpret1/1
  reinterpret1/1 -> concatenate/1
  in2/1 -> reinterpret2/1
  reinterpret2/1 -> concatenate/2

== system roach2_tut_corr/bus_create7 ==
  in1 : Inport
  in2 : Inport  Port=2
  concatenate : xbsIndex_r4/Concat  num_inputs=2  dbl_ovrd=off  block_type=concat
  reinterpret1 : xbsIndex_r4/Reinterpret  force_arith_type=on  arith_type=Unsigned  force_bin_pt=on  bin_pt=0  block_type=reinterpret
  reinterpret2 : xbsIndex_r4/Reinterpret  force_arith_type=on  arith_type=Unsigned  force_bin_pt=on  bin_pt=0  block_type=reinterpret
  bus_out : Outport
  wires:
  concatenate/1 -> bus_out/1
  in1/1 -> reinterpret1/1
  reinterpret1/1 -> concatenate/1
  in2/1 -> reinterpret2/1
  reinterpret2/1 -> concatenate/2

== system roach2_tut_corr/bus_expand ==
  bus_in : Inport
  reinterpret{1..4} (4 alike) : xbsIndex_r4/Reinterpret  force_arith_type=on  arith_type="Signed  (2's comp)"  force_bin_pt=on  bin_pt=7  block_type=reinterpret
  slice1 : xbsIndex_r4/Slice  nbits=8  boolean_output=off  mode=Upper Bit Location + Width  bit1=-24  base1=MSB of Input  bit0=0  base0=LSB of Input  dbl_ovrd=off  block_type=slice
  slice2 : xbsIndex_r4/Slice  nbits=8  boolean_output=off  mode=Upper Bit Location + Width  bit1=-16  base1=MSB of Input  bit0=0  base0=LSB of Input  dbl_ovrd=off  block_type=slice
  slice3 : xbsIndex_r4/Slice  nbits=8  boolean_output=off  mode=Upper Bit Location + Width  bit1=-8  base1=MSB of Input  bit0=0  base0=LSB of Input  dbl_ovrd=off  block_type=slice
  slice4 : xbsIndex_r4/Slice  nbits=8  boolean_output=off  mode=Upper Bit Location + Width  bit1=0  base1=MSB of Input  bit0=0  base0=LSB of Input  dbl_ovrd=off  block_type=slice
  msb_out4 : Outport
  out3 : Outport  Port=2
  out2 : Outport  Port=3
  lsb_out1 : Outport  Port=4
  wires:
  bus_in/1 -> slice4/1, slice3/1, slice2/1, slice1/1
  slice4/1 -> reinterpret4/1
  reinterpret4/1 -> msb_out4/1
  slice3/1 -> reinterpret3/1
  reinterpret3/1 -> out3/1
  slice2/1 -> reinterpret2/1
  reinterpret2/1 -> out2/1
  slice1/1 -> reinterpret1/1
  reinterpret1/1 -> lsb_out1/1

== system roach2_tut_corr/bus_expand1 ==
  bus_in : Inport
  reinterpret{1..4} (4 alike) : xbsIndex_r4/Reinterpret  force_arith_type=on  arith_type="Signed  (2's comp)"  force_bin_pt=on  bin_pt=7  block_type=reinterpret
  slice1 : xbsIndex_r4/Slice  nbits=8  boolean_output=off  mode=Upper Bit Location + Width  bit1=-24  base1=MSB of Input  bit0=0  base0=LSB of Input  dbl_ovrd=off  block_type=slice
  slice2 : xbsIndex_r4/Slice  nbits=8  boolean_output=off  mode=Upper Bit Location + Width  bit1=-16  base1=MSB of Input  bit0=0  base0=LSB of Input  dbl_ovrd=off  block_type=slice
  slice3 : xbsIndex_r4/Slice  nbits=8  boolean_output=off  mode=Upper Bit Location + Width  bit1=-8  base1=MSB of Input  bit0=0  base0=LSB of Input  dbl_ovrd=off  block_type=slice
  slice4 : xbsIndex_r4/Slice  nbits=8  boolean_output=off  mode=Upper Bit Location + Width  bit1=0  base1=MSB of Input  bit0=0  base0=LSB of Input  dbl_ovrd=off  block_type=slice
  msb_out4 : Outport
  out3 : Outport  Port=2
  out2 : Outport  Port=3
  lsb_out1 : Outport  Port=4
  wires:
  bus_in/1 -> slice4/1, slice3/1, slice2/1, slice1/1
  slice4/1 -> reinterpret4/1
  reinterpret4/1 -> msb_out4/1
  slice3/1 -> reinterpret3/1
  reinterpret3/1 -> out3/1
  slice2/1 -> reinterpret2/1
  reinterpret2/1 -> out2/1
  slice1/1 -> reinterpret1/1
  reinterpret1/1 -> lsb_out1/1

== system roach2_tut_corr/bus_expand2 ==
  bus_in : Inport
  reinterpret{1..4} (4 alike) : xbsIndex_r4/Reinterpret  force_arith_type=on  arith_type="Signed  (2's comp)"  force_bin_pt=on  bin_pt=7  block_type=reinterpret
  slice1 : xbsIndex_r4/Slice  nbits=8  boolean_output=off  mode=Upper Bit Location + Width  bit1=-24  base1=MSB of Input  bit0=0  base0=LSB of Input  dbl_ovrd=off  block_type=slice
  slice2 : xbsIndex_r4/Slice  nbits=8  boolean_output=off  mode=Upper Bit Location + Width  bit1=-16  base1=MSB of Input  bit0=0  base0=LSB of Input  dbl_ovrd=off  block_type=slice
  slice3 : xbsIndex_r4/Slice  nbits=8  boolean_output=off  mode=Upper Bit Location + Width  bit1=-8  base1=MSB of Input  bit0=0  base0=LSB of Input  dbl_ovrd=off  block_type=slice
  slice4 : xbsIndex_r4/Slice  nbits=8  boolean_output=off  mode=Upper Bit Location + Width  bit1=0  base1=MSB of Input  bit0=0  base0=LSB of Input  dbl_ovrd=off  block_type=slice
  msb_out4 : Outport
  out3 : Outport  Port=2
  out2 : Outport  Port=3
  lsb_out1 : Outport  Port=4
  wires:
  bus_in/1 -> slice4/1, slice3/1, slice2/1, slice1/1
  slice4/1 -> reinterpret4/1
  reinterpret4/1 -> msb_out4/1
  slice3/1 -> reinterpret3/1
  reinterpret3/1 -> out3/1
  slice2/1 -> reinterpret2/1
  reinterpret2/1 -> out2/1
  slice1/1 -> reinterpret1/1
  reinterpret1/1 -> lsb_out1/1

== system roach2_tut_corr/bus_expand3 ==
  bus_in : Inport
  reinterpret{1..4} (4 alike) : xbsIndex_r4/Reinterpret  force_arith_type=on  arith_type="Signed  (2's comp)"  force_bin_pt=on  bin_pt=7  block_type=reinterpret
  slice1 : xbsIndex_r4/Slice  nbits=8  boolean_output=off  mode=Upper Bit Location + Width  bit1=-24  base1=MSB of Input  bit0=0  base0=LSB of Input  dbl_ovrd=off  block_type=slice
  slice2 : xbsIndex_r4/Slice  nbits=8  boolean_output=off  mode=Upper Bit Location + Width  bit1=-16  base1=MSB of Input  bit0=0  base0=LSB of Input  dbl_ovrd=off  block_type=slice
  slice3 : xbsIndex_r4/Slice  nbits=8  boolean_output=off  mode=Upper Bit Location + Width  bit1=-8  base1=MSB of Input  bit0=0  base0=LSB of Input  dbl_ovrd=off  block_type=slice
  slice4 : xbsIndex_r4/Slice  nbits=8  boolean_output=off  mode=Upper Bit Location + Width  bit1=0  base1=MSB of Input  bit0=0  base0=LSB of Input  dbl_ovrd=off  block_type=slice
  msb_out4 : Outport
  out3 : Outport  Port=2
  out2 : Outport  Port=3
  lsb_out1 : Outport  Port=4
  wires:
  bus_in/1 -> slice4/1, slice3/1, slice2/1, slice1/1
  slice4/1 -> reinterpret4/1
  reinterpret4/1 -> msb_out4/1
  slice3/1 -> reinterpret3/1
  reinterpret3/1 -> out3/1
  slice2/1 -> reinterpret2/1
  reinterpret2/1 -> out2/1
  slice1/1 -> reinterpret1/1
  reinterpret1/1 -> lsb_out1/1

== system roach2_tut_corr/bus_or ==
  In1 : Inport
  Logical5 : xbsIndex_r4/Logical  logical_function=OR  inputs=4  en=off  latency=2  precision=Full  arith_type=Unsigned  n_bits=16  bin_pt=0  align_bp=on  dbl_ovrd=off  block_type=logical
  bus_expand4 : Subsystem  AncestorBlock=casper_library_flow_control/bus_expand
  Out1 : Outport
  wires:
  Logical5/1 -> Out1/1
  In1/1 -> bus_expand4/1(bus_in)
  bus_expand4/2(out3) -> Logical5/2
  bus_expand4/3(out2) -> Logical5/3
  bus_expand4/4(lsb_out1) -> Logical5/4
  bus_expand4/1(msb_out4) -> Logical5/1
